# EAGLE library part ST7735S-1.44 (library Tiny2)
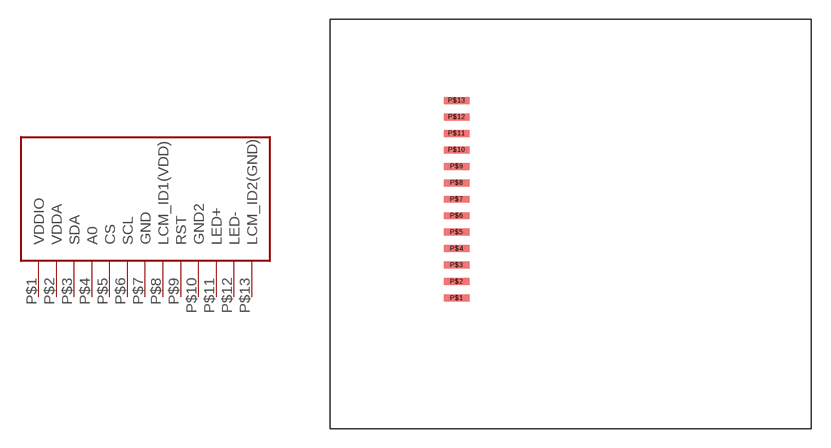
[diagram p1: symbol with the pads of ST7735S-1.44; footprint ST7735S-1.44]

Designator prefix -

## ST7735S-1.44  [ST7735S-1.44]
P$1  VDDIO
P$2  VDDA
P$3  SDA
P$4  A0
P$5  CS
P$6  SCL
P$7  GND
P$8  LCM_ID1(VDD)
P$9  RST
P$10  GND2
P$11  LED+
P$12  LED-
P$13  LCM_ID2(GND)

## Footprint ST7735S-1.44 (pad centres in mm)
smd 2 x 0.55: P$1 -9,-5.85; P$2 -9,-4.55; P$3 -9,-3.25; P$4 -9,-1.95; P$5 -9,-0.65; P$6 -9,0.65; P$7 -9,1.95; P$8 -9,3.25; P$9 -9,4.55; P$10 -9,5.85; P$11 -9,7.15; P$12 -9,8.45; P$13 -9,9.75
